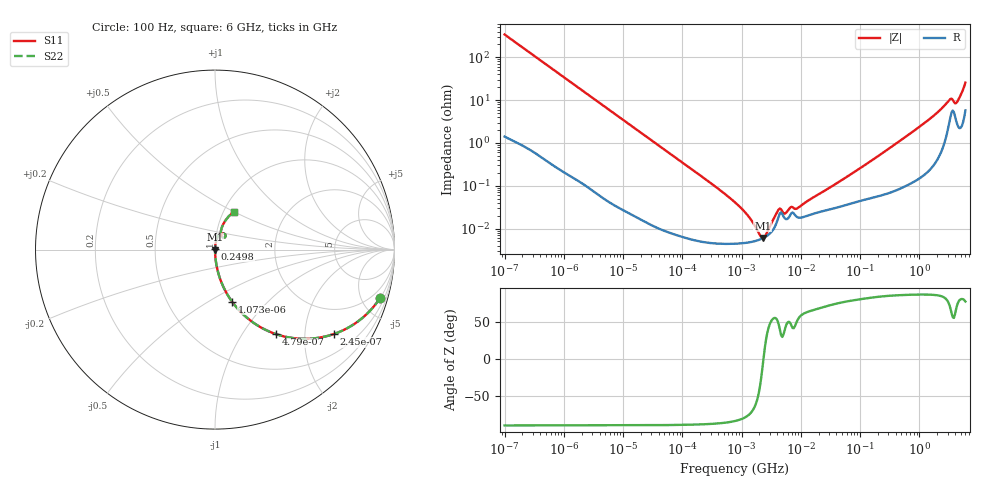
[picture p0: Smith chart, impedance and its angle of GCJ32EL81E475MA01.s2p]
!Murata Part Number: GCJ32EL81E475MA01
!These Parameters are Measured in Series Mode Connection
!Data Generated on Mar 13, 2026
!  o--ll--o
!Port1  Port2
!  o------o
!Operation Temp=25[degC], DC Bias Voltage=0[V]
!Freq. Start=100[Hz] Stop=6[GHz] 401[Steps]
# Hz S RI R 50
!Freq.(Hz) S11(Real) S11(Imag) S21(Real) S21(Imag) S12(Real) S12(Imag) S22(Real) S22(Imag)
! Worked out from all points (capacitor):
!   401 points, 100 Hz to 6 GHz, reference 50 ohm
!   read as one part in series: C = 4.65 uF near 109 Hz
!   lowest |Z| = 6 mohm at 2.269 MHz (marker M1)
!   series resonance near 2.342 MHz, so ESL is about 990 pH
!   S11 on the Smith chart (normalised r, x): 100 Hz: 1.03, -6.84; 245 Hz: 1.01, -2.80; 479 Hz: 1.01, -1.43; 1.073 kHz: 1.00, -0.64; 249.8 MHz: 1.00, +0.01; 6 GHz: 1.12, +0.50
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100  0.9203 -0.2688  0.0797 0.2688  0.0797 0.2688  0.9203 -0.2688
245  0.6615 -0.4706  0.3385 0.4706  0.3385 0.4706  0.6615 -0.4706
479  0.3406 -0.4711  0.6594 0.4711  0.6594 0.4711  0.3406 -0.4711
1073  0.095 -0.2902  0.905 0.2902  0.905 0.2902  0.095 -0.2902
2008  0.0298 -0.1668  0.9702 0.1668  0.9702 0.1668  0.0298 -0.1668
6433  0.00328 -0.0538  0.9967 0.0538  0.9967 0.0538  0.00328 -0.0538
40335  0.000175 -0.00868  0.9998 0.00868  0.9998 0.00868  0.000175 -0.00868
774597  4.43e-05 -0.000407  1 0.000407  1 0.000407  4.43e-05 -0.000407
1734173  5.16e-05 -9.36e-05  0.9999 9.36e-05  0.9999 9.36e-05  5.16e-05 -9.36e-05
2268635  5.92e-05 -9.9e-06  0.9999 9.9e-06  0.9999 9.9e-06  5.92e-05 -9.9e-06
2967816  7.54e-05 7.76e-05  0.9999 -7.76e-05  0.9999 -7.76e-05  7.54e-05 7.76e-05
4246196  0.000196 0.000202  0.9998 -0.000202  0.9998 -0.000202  0.000196 0.000202
5554849  0.000167 0.000158  0.9998 -0.000158  0.9998 -0.000158  0.000167 0.000158
6948629  0.00023 0.000226  0.9998 -0.000226  0.9998 -0.000226  0.00023 0.000226
9090158  0.000181 0.000249  0.9998 -0.000249  0.9998 -0.000249  0.000181 0.000249
1.555665e7  0.000217 0.000468  0.9998 -0.000468  0.9998 -0.000468  0.000217 0.000468
2.497637e8  0.000652 0.00601  0.9993 -0.00601  0.9993 -0.00601  0.000652 0.00601
3.124326e8  0.000735 0.00747  0.9993 -0.00747  0.9993 -0.00747  0.000735 0.00747
1.497423e9  0.00364 0.036  0.9964 -0.036  0.9964 -0.036  0.00364 0.036
3.205649e9  0.0372 0.0903  0.9628 -0.0903  0.9628 -0.0903  0.0372 0.0903
4.193612e9  0.0374 0.0733  0.9626 -0.0733  0.9626 -0.0733  0.0374 0.0733
6e9  0.1044 0.2115  0.8956 -0.2115  0.8956 -0.2115  0.1044 0.2115
